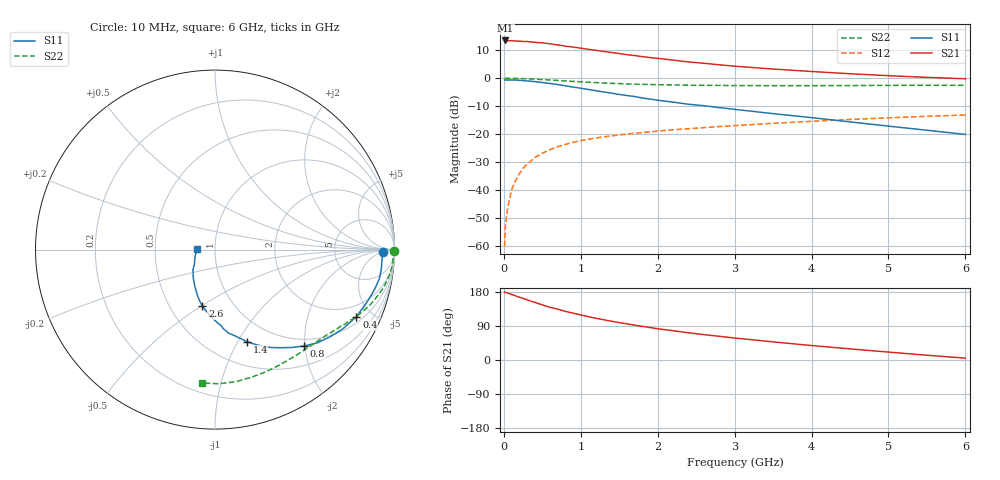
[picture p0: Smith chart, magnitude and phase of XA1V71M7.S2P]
! SIEMENS Discrete & RF Semiconductors
! BFY180
! Si NPN RF Bipolar Junction Transistor in MICRO-X
! VCE = 1.75 V  IC = 1.7 mA
! Common Emitter S-Parameters:  May  1997
# GHz  S  MA  R  50
!  f  S11  S21  S12  S22
! GHz  MAG  ANG  MAG  ANG  MAG  ANG  MAG  ANG
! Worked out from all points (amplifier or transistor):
!   36 points, 10 MHz to 6 GHz, reference 50 ohm
!   highest |S21| = 13.5 dB at 20 MHz (marker M1)
!   |S21| within 3 dB of that: start of sweep to 1.061 GHz
!   unconditionally stable (mu >= 1): 2.665 GHz to end of sweep
!   at 250 MHz: K = 0.13, MSG = 22.7 dB, |S12| = -32.2 dB
!   at 1.4 GHz: K = 0.69, MSG = 14.9 dB, |S12| = -20.6 dB
!   at 6 GHz: K = 1.09, MAG = 4.6 dB, |S12| = -13.1 dB
!   S11 on the Smith chart (normalised r, x): 10 MHz: 29, -5; 400 MHz: 1.30, -4.04; 800 MHz: 0.86, -1.98; 1.4 GHz: 0.75, -1.09; 2.6 GHz: 0.72, -0.51; 6 GHz: 0.82, +0.01
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0.01  0.9358 -0.7  4.67 179.4  0.001 93.6  0.9946 -0.3
0.02  0.9325 -1.5  4.729 178.5  0.0023 91.9  0.9999 -0.6
0.05  0.9325 -3.2  4.642 176.6  0.0049 87.7  0.995 -1.6
0.1  0.9329 -6.7  4.684 173.1  0.01 87.6  0.9928 -3.3
0.15  0.9301 -9.9  4.634 169.5  0.0147 85.0  0.9929 -4.9
0.3  0.8946 -19.4  4.522 158.8  0.0289 77.7  0.9762 -9.6
0.4  0.8717 -25.4  4.381 152.2  0.0379 74.0  0.9636 -12.5
0.5  0.8386 -31.7  4.277 145.5  0.0458 70.0  0.9467 -15.2
0.6  0.8047 -37.1  4.122 139.0  0.0529 66.9  0.9297 -17.8
0.8  0.7315 -47.2  3.742 128.3  0.0658 60.9  0.8938 -22.4
1  0.6616 -55.7  3.448 118.8  0.0769 56.3  0.8628 -26.4
1.1  0.6295 -60.1  3.286 114.4  0.0811 54.4  0.8472 -28.0
1.4  0.5422 -70.9  2.879 102.3  0.0934 49.4  0.8105 -33.0
1.5  0.5139 -74.2  2.759 98.5  0.0971 48.1  0.8008 -34.4
1.8  0.4437 -83.9  2.433 88.8  0.1074 45.3  0.778 -38.7
2  0.4043 -88.6  2.265 82.5  0.1137 43.2  0.7666 -41.4
2.2  0.3745 -93.4  2.107 77.2  0.12 41.4  0.7592 -44.1
2.6  0.3233 -102.5  1.851 66.9  0.1312 38.5  0.7467 -49.3
3.5  0.233 -118.9  1.459 47.8  0.1565 32.4  0.7365 -60.8
4.5  0.166 -137.6  1.203 29.3  0.1834 25.2  0.7398 -74.1
5.5  0.1177 -161.0  1.037 12.6  0.2087 17.4  0.7477 -88.3
6  0.0992 177.3  0.978 4.9  0.2202 13.2  0.747 -95.4
